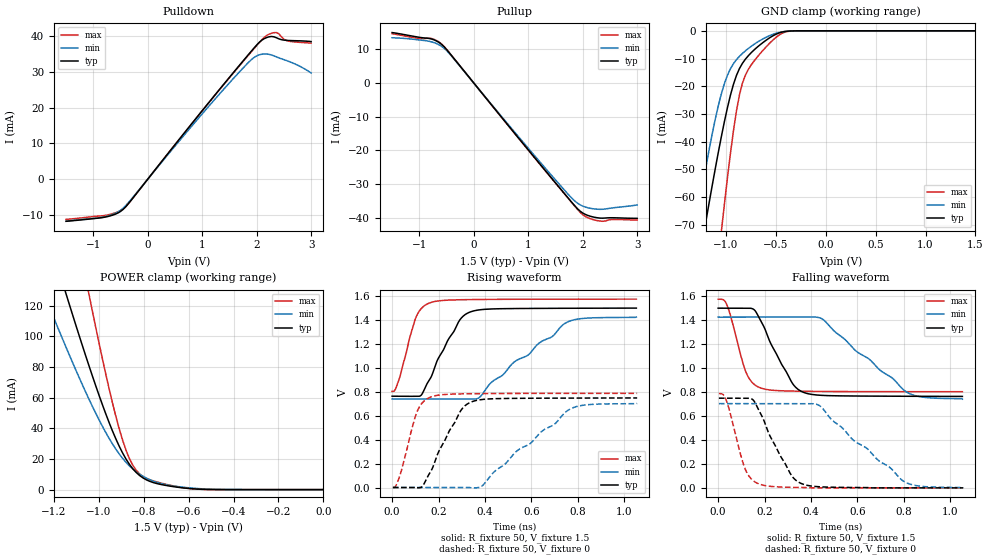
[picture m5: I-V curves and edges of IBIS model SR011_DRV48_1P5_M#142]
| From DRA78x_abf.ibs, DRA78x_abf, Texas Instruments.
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| Model based on original model for DDR_SEIOPB_V
|   Sub model SR011_DRV48_1P5
[model]   SR011_DRV48_1P5_M#142
|[Description]  [1.5V-I/O-X-X]
|   , ,
|[Input Load]
|[Output Drive]
|Voltage   1.5V
|Mode   I/O
Model_type   I/O
Polarity   Non-Inverting
Enable   Active-Low
Vinl =  0.65
Vinh =  0.85
Cref =  15.0000pF
Rref =  100.0000M
Vref =  0V
Vmeas =  0.75
C_comp   2p   2p   2p
[Model Spec]
Vinl   0.65   0.6125   0.6875
Vinh   0.85   0.8125   0.8875
[Receiver Thresholds]
Tslew_ac = 0.5n
Vth = 0.75
Vth_max = 0.7875
Vth_min = 0.675
Vinh_ac = 0.175
Vinh_dc = 0.1
Vinl_ac = -0.175
Vinl_dc = -0.1
[Temperature Range]   25   125   -40
[Voltage Range]   1.5   1.425   1.575
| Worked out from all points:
|   slope of the pulldown table from 0 to 0.225 V, typ, clamps not added: 51.5 ohm
|   slope of the pullup table from 0 to 0.225 V, typ, clamps not added: 50.1 ohm
|   GND clamp passes 1 mA (typ) near -0.48 V on its own axis
|   POWER clamp passes 1 mA (typ) near -0.62 V on its own axis
|   rising waveform, R_fixture 50, V_fixture 1.5: 20-80 % time 114ps typ, 276ps min, 64.3ps max; typ from 0.763 V to 1.5 V
|   rising waveform, R_fixture 50, V_fixture 0: 20-80 % time 113ps typ, 271ps min, 64.6ps max; typ from 0 V to 0.749 V
|   falling waveform, R_fixture 50, V_fixture 1.5: 20-80 % time 114ps typ, 258ps min, 66ps max; typ from 1.5 V to 0.763 V
|   falling waveform, R_fixture 50, V_fixture 0: 20-80 % time 114ps typ, 263ps min, 65.2ps max; typ from 0.749 V to 0 V
[POWER_clamp]
-1.5V     302.8mA    223.9mA    484.4mA
-1.242V   174.3mA    127.3mA    279.1mA
-1.136V   123.3mA    89.68mA    196.8mA
-1.045V   81.65mA    59.62mA    128.8mA
-1.03V    75mA       54.92mA    117.8mA
-939.4mV  38.44mA    29.91mA    56.84mA
-893.9mV  23.93mA    20.41mA    32.31mA
-848.5mV  13.61mA    13.43mA    15.91mA
-803mV    7.623mA    8.663mA    8.564mA
-712.1mV  3.022mA    3.561mA    3.877mA
-575.8mV  470.5uA    872uA      449uA
0V        112.6nA    435.6nA    613.8nA
[Pulldown]
-1.5V     -11.81mA   -11.79mA   -11.27mA
-727.3mV  -10.45mA   -10.3mA    -10mA
-545.5mV  -9.463mA   -9.189mA   -9.136mA
-409.1mV  -7.817mA   -7.49mA    -7.751mA
1.227V    23.47mA    22.31mA    23.4mA
1.818V    34.37mA    32.24mA    34.22mA
2V        37.61mA    34.55mA    37.45mA
2.136V    39.37mA    35.1mA     39.71mA
2.318V    39.9mA     34.55mA    41.07mA
2.409V    39.32mA    34mA       40.72mA
2.545V    38.91mA    33.26mA    38.88mA
3V        38.57mA    29.76mA    38.14mA
[Pullup]
-1.5V     14.98mA    13.43mA    14.66mA
-1V       13.57mA    12.78mA    13.25mA
-772.7mV  13.05mA    12.2mA     13.19mA
-590.9mV  11.46mA    10.89mA    11.59mA
-409.1mV  8.169mA    8.001mA    8.195mA
1.409V    -27.86mA   -27.07mA   -27.94mA
1.773V    -34.91mA   -33.72mA   -35mA
1.909V    -37.4mA    -35.72mA   -37.61mA
2.045V    -38.99mA   -36.82mA   -39.6mA
2.273V    -40.02mA   -37.48mA   -40.87mA
2.591V    -40.02mA   -37mA      -40.5mA
3V        -40.19mA   -36.21mA   -40.69mA
[GND_clamp]
-1.5V     -133.6mA   -115.7mA   -234.3mA
-1.288V   -87.29mA   -67.59mA   -156.8mA
-1.197V   -68.11mA   -48.64mA   -124.4mA
-1.045V   -38.25mA   -22.77mA   -72.51mA
-1.015V   -32.88mA   -19.1mA    -62.74mA
-954.5mV  -23.3mA    -13.72mA   -44.4mA
-863.6mV  -13.6mA    -9.192mA   -23.11mA
-803mV    -10.18mA   -7.193mA   -15.89mA
-681.8mV  -5.771mA   -4.027mA   -9.287mA
-500mV    -1.264mA   -914.7uA   -2.429mA
-348.5mV  -52.39uA   -75.11uA   -85.87uA
1.5V      112.6nA    528.1nA    514.5nA
[Ramp]
dV/dt_f 0.44249778/0.11369971n 0.41135398/0.25813314n 0.46375208/65.983832p
dV/dt_r 0.45073521/0.11305148n 0.42376072/0.27205694n  0.4736695/64.702818p
R_load = 50
[Rising Waveform]
R_fixture = 50
V_fixture = 1.5
V_fixture_min = 1.425
V_fixture_max = 1.575
0s        763.3mV    740.8mV    803.4mV
31.78ps   762.6mV    740.7mV    914.4mV
102.5ps   761.8mV    740.7mV    1.421V
126.6ps   774.5mV    740.7mV    1.498V
159.8ps   896.6mV    740.7mV    1.542V
287.1ps   1.387V     740.6mV    1.57V
339.5ps   1.47V      738.8mV    1.571V
377.1ps   1.486V     754.1mV    1.572V
754.1ps   1.499V     1.382V     1.575V
1.053ns   1.5V       1.425V     1.575V
[Rising Waveform]
R_fixture = 50
V_fixture = 0
V_fixture_min = 0
V_fixture_max = 0
3.401ps   0V         0V         0V
35.01ps   0V         0V         107.5mV
107.3ps   -2.06mV    0V         632.7mV
131.1ps   11.19mV    0V         710mV
166.2ps   133.6mV    0V         756.5mV
292.3ps   631.7mV    0V         782.8mV
346.2ps   718.9mV    -2.576mV   784.3mV
387.7ps   735.8mV    13.29mV    785.1mV
767.7ps   747.6mV    656.5mV    787.1mV
1.056ns   748.7mV    703.3mV    787.3mV
[Falling Waveform]
R_fixture = 50
V_fixture = 1.5
V_fixture_min = 1.425
V_fixture_max = 1.575
0s        1.5V       1.425V     1.575V
39.87ps   1.5V       1.425V     1.517V
125.3ps   1.501V     1.425V     942.6mV
156.4ps   1.485V     1.425V     862.5mV
183.1ps   1.396V     1.425V     833.9mV
316.5ps   883.7mV    1.425V     807.7mV
369.2ps   796.5mV    1.425V     806.1mV
451.7ps   771.6mV    1.406V     804.6mV
819.1ps   764.5mV    792.4mV    802.7mV
1.053ns   763.3mV    740.8mV    802.5mV
[Falling Waveform]
R_fixture = 50
V_fixture = 0
V_fixture_min = 0
V_fixture_max = 0
3.401ps   748.7mV    703.3mV    787.3mV
37.86ps   748.9mV    703.3mV    716.4mV
118.5ps   748.8mV    703.3mV    148.2mV
150.1ps   735.1mV    703.3mV    61.4mV
174.6ps   651.2mV    703.3mV    33.55mV
310.7ps   120.5mV    703.2mV    4.574mV
361.7ps   33.68mV    703.4mV    2.869mV
439.6ps   8.661mV    683mV      0V
805.8ps   0V         47.94mV    0V
1.056ns   0V         0V         0V
